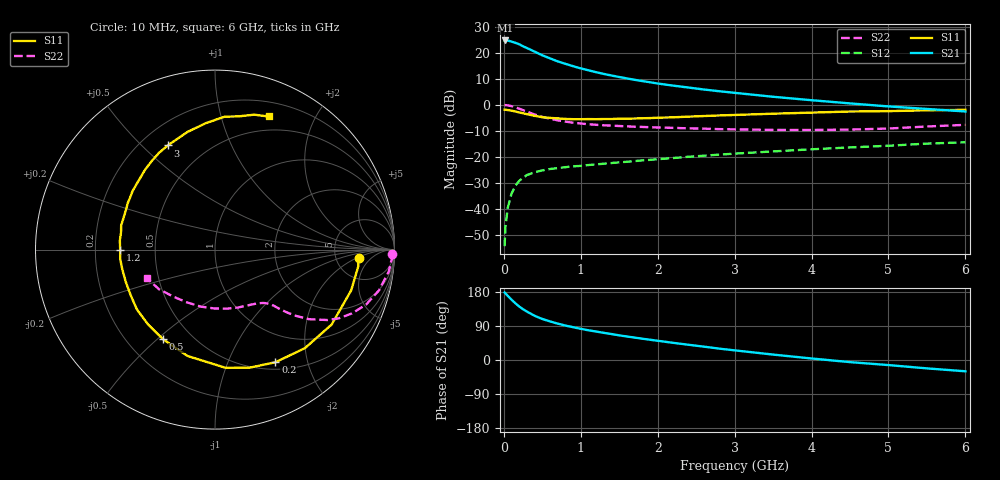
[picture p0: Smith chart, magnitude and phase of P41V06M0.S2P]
! SIEMENS Small Signal Semiconductors
! BFP182
! Si NPN RF Bipolar Junction Transistor in SOT143
! VCE = 1 V  IC = 6 mA
! Common Emitter S-Parameters:  March  1996
# GHz  S  MA  R  50
!  f  S11  S21  S12  S22
! GHz  MAG  ANG  MAG  ANG  MAG  ANG  MAG  ANG
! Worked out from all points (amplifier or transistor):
!   36 points, 10 MHz to 6 GHz, reference 50 ohm
!   highest |S21| = 24.8 dB at 20 MHz (marker M1)
!   |S21| within 3 dB of that: start of sweep to 306.6 MHz
!   unconditionally stable (mu >= 1): 1.334 GHz to end of sweep
!   at 250 MHz: K = 0.26, MSG = 25.3 dB, |S12| = -28.1 dB
!   at 1.4 GHz: K = 1.03, MAG = 15.8 dB, |S12| = -22.4 dB
!   at 6 GHz: K = 1.02, MAG = 5.1 dB, |S12| = -14.4 dB
!   S11 on the Smith chart (normalised r, x): 10 MHz: 8.49, -2.26; 200 MHz: 0.59, -1.50; 500 MHz: 0.35, -0.52; 1.2 GHz: 0.31, -0.00; 3 GHz: 0.31, +0.60; 6 GHz: 0.35, +1.42
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0.01  0.802 -3.4  17.26 178.2  0.0019 84.8  0.985 -1.4
0.02  0.8036 -6.7  17.3 176.2  0.0044 85.3  0.9866 -2.9
0.05  0.7919 -16.7  17.27 169.4  0.0103 83.6  0.9758 -7.2
0.1  0.7725 -32.7  16.46 159.1  0.0195 73.3  0.9414 -14.0
0.15  0.7433 -47.6  15.59 149.7  0.0277 66.1  0.8958 -20.0
0.2  0.7122 -61.8  14.62 141.1  0.0344 60.1  0.8417 -25.0
0.25  0.6854 -73.8  13.36 133.8  0.0394 54.9  0.7882 -29.1
0.3  0.6612 -84.9  12.38 127.8  0.0445 51.0  0.7384 -32.1
0.4  0.6121 -104.5  10.54 116.6  0.0502 44.6  0.6519 -36.5
0.5  0.5772 -120.1  8.968 108.3  0.0546 40.5  0.5852 -39.2
0.6  0.5593 -131.8  7.83 101.8  0.058 38.0  0.5382 -40.9
0.7  0.5481 -142.5  6.844 96.0  0.0605 36.7  0.5025 -42.1
0.9  0.5286 -160.1  5.54 86.6  0.0654 34.8  0.452 -43.7
1.1  0.5308 -174.4  4.613 78.4  0.0693 34.3  0.4224 -45.6
1.2  0.5282 -179.8  4.24 75.1  0.0712 33.6  0.4117 -46.5
1.7  0.544 155.5  3.024 59.1  0.0824 34.0  0.3783 -52.4
2.2  0.5737 137.7  2.339 45.3  0.0944 33.3  0.3601 -60.5
3  0.6371 114.4  1.699 25.5  0.1147 30.2  0.3366 -77.5
3.5  0.6736 103.1  1.426 14.3  0.1267 27.5  0.3282 -90.2
4.5  0.7421 85.9  1.063 -5.6  0.1512 21.5  0.3332 -118.1
5.5  0.7828 73.8  0.832 -22.1  0.179 15.2  0.3821 -144.7
6  0.7993 68.1  0.743 -29.8  0.19 10.7  0.4113 -157.0
